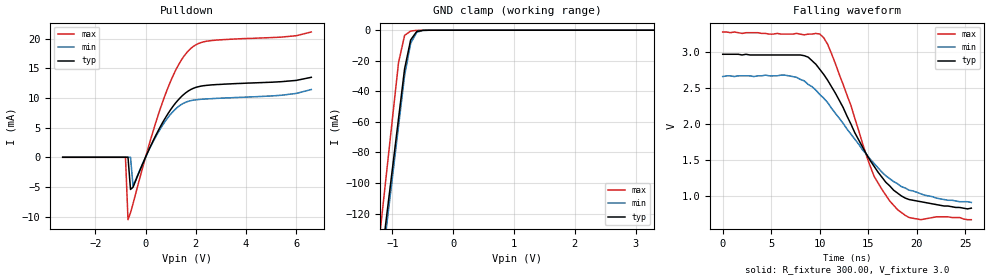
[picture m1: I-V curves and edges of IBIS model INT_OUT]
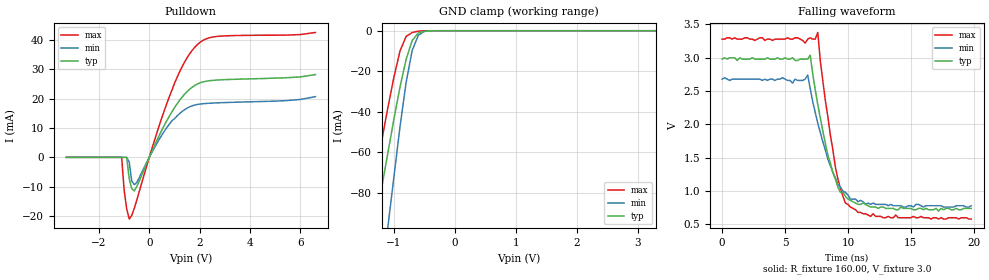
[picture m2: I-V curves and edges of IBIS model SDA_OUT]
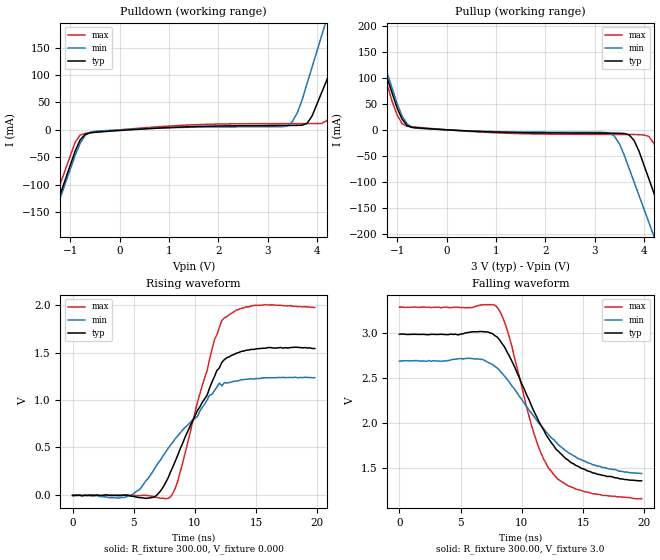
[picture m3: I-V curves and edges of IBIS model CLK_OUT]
| IBIS file 8564nb3v.ibs
[IBIS ver]   3.2
[File name]   8564nb3v.ibs
[File Rev]   1.0
[Date]   Jan 22, 2008
[Source]   This file orginated at EPSON TOYOCOM Corp.
[Copyright]   Copyright EPSON TOYOCOM Corp. 2008
|   Component 8564nb3v
[Component]   8564nb3v
[Manufacturer]   EPSON TOYOCOM
[Package]
| variable   typ   min   max
R_pkg   87m   NA   NA
L_pkg   10nH   NA   NA
C_pkg   206fF   NA   NA
[Pin]  signal_name   model_name   R_pin   L_pin   C_pin
1   /INT   INT_OUT
2   GND   GND
|3   GND
|4   NC
5   SDA   SDA_OUT
6   SCL   SCL_IN
7   CLKOUT   CLK_OUT
8   VDD   POWER
9   CLKOE   OE_IN
|10   NC
|11   NC
|12   NC
|13   NC
|14   NC
|15   NC
|16   NC
|17   NC
|18   NC
|19   NC
|20   NC
|21   NC
|22   NC
5T   SDA   SDA_IN
| Models and submodels in the file (6): INT_OUT (Open_drain), SDA_OUT (Open_drain), CLK_OUT (Output), SCL_IN (Input), OE_IN (Input), SDA_IN (Input)
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|   Model OUTPUT
[Model]   INT_OUT
Model_type   Open_drain
Polarity   Non-Inverting
C_comp   5pF   5pF   5pF
[Temperature Range]   25.00   85.00   -40.000
[Voltage Range]   3.0V   2.7V   3.3V
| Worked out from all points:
|   slope of the pulldown table from 0 to 0.45 V, typ, clamps not added: 112 ohm
|   GND clamp passes 1 mA (typ) near -0.60 V on its own axis
|   falling waveform, R_fixture 300.00, V_fixture 3.0: 20-80 % time 5.31ns typ, 6.27ns min, 4.13ns max; typ from 2.97 V to 0.83 V
[Pulldown]
| voltage   I(typ)   I(min)   I(max)
-3.3V     0A         0A         0A
-800mV    0A         0A         0A
-700mV    0A         0A         -10.53mA
-600mV    -5.43mA    0A         -9.37mA
-500mV    -5.05mA    -4.83mA    -7.84mA
200mV     1.89mA     1.79mA     2.99mA
700mV     6.02mA     5.56mA     9.59mA
1.2V      9.19mA     8.17mA     14.7mA
1.7V      11.18mA    9.44mA     17.95mA
2.4V      12.12mA    9.84mA     19.56mA
5.4V      12.75mA    10.46mA    20.27mA
6.6V      13.49mA    11.43mA    21.14mA
[GND_clamp]
| voltage   I(typ)   I(min)   I(max)
-3.3V     -841.3mA   -861.7mA   -899.7mA
-1.2V     -155.9mA   -162.8mA   -131.1mA
-1.1V     -123.2mA   -129.6mA   -94.5mA
-1V       -90.58mA   -96.29mA   -57.9mA
-900mV    -57.94mA   -63.01mA   -21.3mA
-800mV    -25.3mA    -29.73mA   -3.38mA
-700mV    -6.32mA    -8.59mA    -540uA
-600mV    -840uA     -1.34mA    -90uA
-500mV    -90uA      -130uA     -10uA
3.3V      0A         0A         0A
[Ramp]
| variable   typ   min   max
dV/dt_r 1.41/8.4n   1.19/8.0n   1.69/8.8n
dV/dt_f 1.29/5.2n   1.06/6.4n   1.57/4.4n
R_load = 300.00
[Falling Waveform]
R_fixture = 300.00
V_fixture = 3.0
V_fixture_min = 2.7
V_fixture_max = 3.3
| time   V(typ)   V(min)   V(max)
0s        2.97V      2.66V      3.28V
6.4ns     2.96V      2.68V      3.25V
8.8ns     2.93V      2.55V      3.25V
10ns      2.76V      2.41V      3.25V
10.8ns    2.61V      2.3V       3.11V
11.6ns    2.43V      2.15V      2.84V
15.6ns    1.41V      1.45V      1.27V
17.2ns    1.14V      1.24V      930mV
19.2ns    950mV      1.08V      700mV
25.6ns    830mV      910mV      670mV
[Model]   SDA_OUT
Model_type   Open_drain
Polarity   Non-Inverting
C_comp   5pF   5pF   5pF
[Temperature Range]   25.00   85.00   -40.000
[Voltage Range]   3.0V   2.7V   3.3V
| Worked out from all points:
|   slope of the pulldown table from 0 to 0.45 V, typ, clamps not added: 53.7 ohm
|   GND clamp passes 1 mA (typ) near -0.59 V on its own axis
|   falling waveform, R_fixture 160.00, V_fixture 3.0: 20-80 % time 1.59ns typ, 1.83ns min, 1.34ns max; typ from 2.98 V to 0.74 V
[Pulldown]
| voltage   I(typ)   I(min)   I(max)
-3.3V     0A         0A         0A
-1.1V     0A         0A         0A
-1V       0A         0A         -11.31mA
-900mV    0A         0A         -17.53mA
-800mV    -7.33mA    -1.57mA    -21.03mA
-700mV    -10.66mA   -8.08mA    -19.81mA
-600mV    -11.43mA   -9.31mA    -17.43mA
800mV     14.1mA     11.37mA    20.79mA
1.4V      21.5mA     16.25mA    32.44mA
1.9V      24.95mA    18mA       38.35mA
2.7V      26.34mA    18.56mA    41.2mA
6.6V      28.2mA     20.68mA    42.55mA
[GND_clamp]
| voltage   I(typ)   I(min)   I(max)
-3.3V     -432.5mA   -643.8mA   -385.8mA
-1.5V     -128.2mA   -196.5mA   -101.6mA
-1.4V     -111.3mA   -171.7mA   -85.82mA
-1.3V     -94.35mA   -146.8mA   -70.03mA
-1.1V     -60.53mA   -97.11mA   -38.16mA
-1V       -43.62mA   -72.26mA   -22.92mA
-900mV    -27.81mA   -47.41mA   -10.03mA
-800mV    -14.16mA   -25.58mA   -2.82mA
-700mV    -4.83mA    -9.74mA    -880uA
-600mV    -1.08mA    -2.27mA    -200uA
-400mV    -70uA      -30uA      0A
3.3V      0A         0A         0A
[Ramp]
| variable   typ   min   max
dV/dt_r 1.32/2.0n   1.20/1.8n   1.50/1.8n
dV/dt_f 1.40/1.6n   1.19/2.0n   1.68/1.4n
R_load = 160.00
[Falling Waveform]
R_fixture = 160.00
V_fixture = 3.0
V_fixture_min = 2.7
V_fixture_max = 3.3
| time   V(typ)   V(min)   V(max)
0s        2.98V      2.68V      3.28V
5.6ns     3V         2.62V      3.28V
6.8ns     2.98V      2.74V      3.28V
7ns       3.04V      2.54V      3.3V
7.6ns     2.3V       2.02V      3.38V
8.2ns     1.72V      1.62V      2.36V
9ns       1.18V      1.2V       1.36V
9.8ns     920mV      980mV      820mV
11.8ns    760mV      800mV      620mV
19.8ns    740mV      780mV      580mV
[Model]   CLK_OUT
Model_type   Output
Polarity   Non-Inverting
Enable   Active-High
Vmeas =   1.50V
C_comp   1.69pF   1.32pF   1.96pF
[Temperature Range]   25.00   85.00   -40.000
[Voltage Range]   3.0V   2.7V   3.3V
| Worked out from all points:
|   slope of the pulldown table from 0 to 0.45 V, typ, clamps not added: 172 ohm
|   slope of the pullup table from 0 to 0.45 V, typ, clamps not added: 198 ohm
|   rising waveform, R_fixture 300.00, V_fixture 0.000: 20-80 % time 3.32ns typ, 4.41ns min, 2.38ns max; typ from -0.004 V to 1.54 V
|   falling waveform, R_fixture 300.00, V_fixture 3.0: 20-80 % time 3.72ns typ, 4.57ns min, 2.68ns max; typ from 2.99 V to 1.36 V
[Pulldown]
| voltage   I(typ)   I(min)   I(max)
-3.3V     -664.4mA   -662.3mA   -624.4mA
-1.6V     -220.8mA   -225.8mA   -197.8mA
-1.5V     -194.8mA   -200.1mA   -172.7mA
-900mV    -38.21mA   -46mA      -22.2mA
-600mV    -5.52mA    -4.34mA    -5.15mA
3.4V      7.99mA     7.06mA     11.32mA
3.6V      8.15mA     30.89mA    11.36mA
3.8V      12.1mA     84.86mA    11.39mA
4.1V      69.21mA    173.6mA    11.74mA
4.6V      179mA      321.4mA    89.51mA
5.1V      288.7mA    469.3mA    180.1mA
6.3V      552.1mA    824.1mA    397.6mA
[Pullup]
| voltage   I(typ)   I(min)   I(max)
-3V       610mA      636.2mA    670.7mA
-1.5V     183.7mA    196.6mA    183.7mA
-1V       41.63mA    50.02mA    28.46mA
-800mV    8.03mA     11.65mA    6.96mA
3.3V      -6.39mA    -6.24mA    -8.85mA
3.5V      -6.57mA    -26.27mA   -8.92mA
3.8V      -20.18mA   -100.1mA   -9.06mA
4.1V      -94.15mA   -177.9mA   -12.56mA
4.2V      -120.8mA   -203.9mA   -25.69mA
4.5V      -200.8mA   -281.7mA   -103.7mA
4.9V      -307.4mA   -385.5mA   -207.7mA
6.6V      -760.7mA   -826.5mA   -649.7mA
[Ramp]
| variable   typ   min   max
dV/dt_r 0.836/3.4n   0.645/4.2n   1.107/2.6n
dV/dt_f 0.995/3.8n   0.768/4.6n   1.293/2.2n
R_load = 300.00
[Rising Waveform]
R_fixture = 300.00
V_fixture = 0.000
| time   V(typ)   V(min)   V(max)
0s        -4.06mV    -9.06mV    -7.81mV
4.8ns     -13.13mV   -1.02mV    -9.61mV
6.8ns     -12.5mV    296.5mV    -27.81mV
8ns       238.1mV    523.4mV    -22.34mV
8.6ns     419mV      621.6mV    146.4mV
10.2ns    888.4mV    824.8mV    970.8mV
11.6ns    1.247V     1.1V       1.638V
12.2ns    1.396V     1.148V     1.837V
14.6ns    1.534V     1.224V     1.992V
19.8ns    1.543V     1.236V     1.975V
[Falling Waveform]
R_fixture = 300.00
V_fixture = 3.0
V_fixture_min = 2.7
V_fixture_max = 3.3
| time   V(typ)   V(min)   V(max)
0s        2.987V     2.689V     3.288V
5.8ns     3.012V     2.72V      3.282V
7.8ns     2.973V     2.632V     3.312V
8.2ns     2.922V     2.582V     3.245V
8.8ns     2.79V      2.488V     3.038V
10.8ns    2.192V     2.111V     1.973V
12.2ns    1.828V     1.871V     1.496V
13ns      1.687V     1.762V     1.374V
14.8ns    1.504V     1.598V     1.256V
19.8ns    1.36V      1.44V      1.162V
